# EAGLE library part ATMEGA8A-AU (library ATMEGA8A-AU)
Programmable Flash
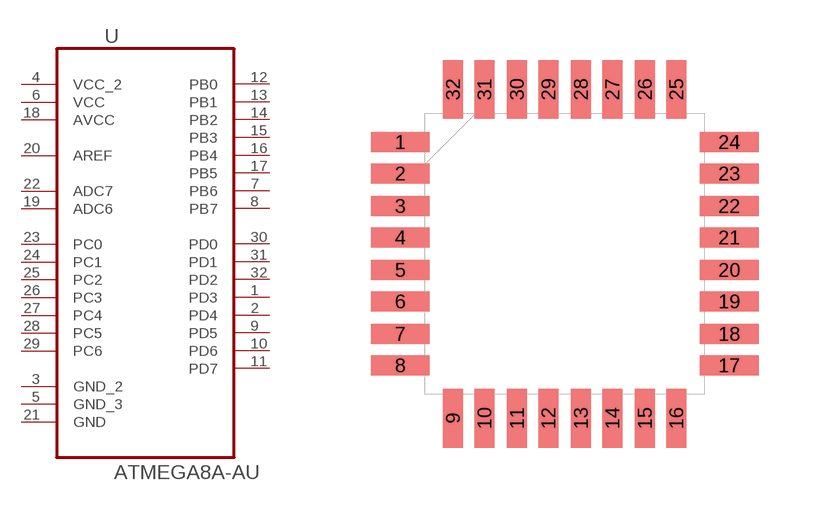
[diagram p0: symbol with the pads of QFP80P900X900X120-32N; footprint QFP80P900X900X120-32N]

Designator prefix U

## ATMEGA8A-AU (Availability: Unavailable; Description: AVR AVR® ATmega Microcontroller IC 8-Bit 16MHz 8KB _4K x 16_ FLASH 32-TQFP _7x7_; MF: Microchip; MP: ATMEGA8A-AU; Package: TQFP-32 Microchip; Price: None)  [QFP80P900X900X120-32N]
1  PD3
2  PD4
3  GND_2  pas
4  VCC_2  pwr
5  GND_3  pas
6  VCC  pwr
7  PB6
8  PB7  pas
9  PD5  pas
10  PD6  pas
11  PD7  pas
12  PB0  pas
13  PB1  pas
14  PB2  pas
15  PB3  pas
16  PB4  pas
17  PB5  pas
18  AVCC  pwr
19  ADC6  in
20  AREF  in
21  GND  pas
22  ADC7  in
23  PC0
24  PC1
25  PC2
26  PC3
27  PC4
28  PC5
29  PC6
30  PD0
31  PD1
32  PD2

## Footprint QFP80P900X900X120-32N (pad centres in mm)
smd 1.473 x 0.508: 1 -4.115,2.794; 2 -4.115,2.007; 3 -4.115,1.194; 4 -4.115,0.406; 5 -4.115,-0.406; 6 -4.115,-1.194; 7 -4.115,-2.007; 8 -4.115,-2.794; 17 4.115,-2.794; 18 4.115,-2.007; 19 4.115,-1.194; 20 4.115,-0.406; 21 4.115,0.406; 22 4.115,1.194; 23 4.115,2.007; 24 4.115,2.794
smd 0.508 x 1.473: 9 -2.794,-4.115; 10 -2.007,-4.115; 11 -1.194,-4.115; 12 -0.406,-4.115; 13 0.406,-4.115; 14 1.194,-4.115; 15 2.007,-4.115; 16 2.794,-4.115; 25 2.794,4.115; 26 2.007,4.115; 27 1.194,4.115; 28 0.406,4.115; 29 -0.406,4.115; 30 -1.194,4.115; 31 -2.007,4.115; 32 -2.794,4.115

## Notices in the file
This work is licensed under a Creative Commons Attribution-ShareAlike 4.0 International License (CC BY-SA) with Design Exception 1.0
